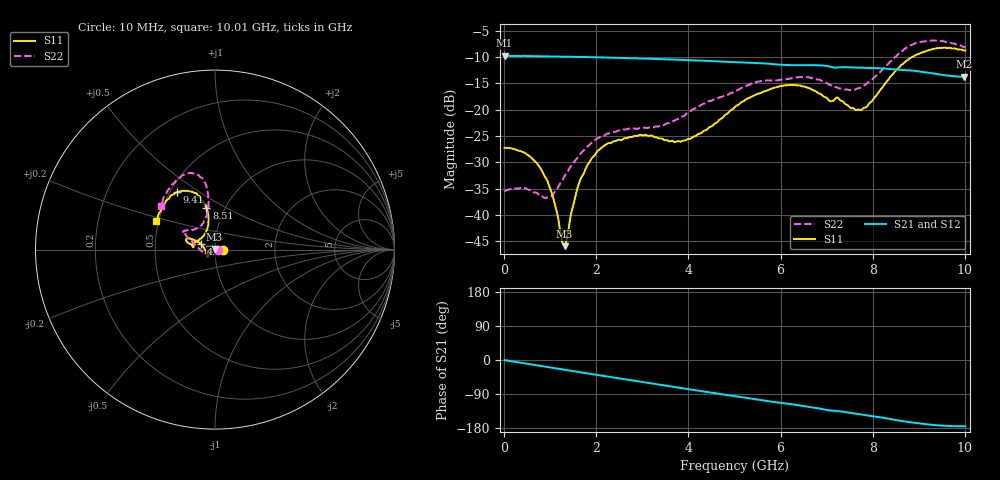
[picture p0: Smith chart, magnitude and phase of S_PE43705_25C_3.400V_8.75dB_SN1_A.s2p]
! Device ID: PE43705
! Serial: 1
! Insertion: A
! Impedance: 50 ohm
! Temp: 25C
! VDD: 3.400V
! Attenuation Step: 8.75dB
#  Hz  S  RI  R  50
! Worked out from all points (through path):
!   401 points, 10 MHz to 10.01 GHz, reference 50 ohm
!   highest |S21| = -9.78 dB at 10 MHz (marker M1); lowest = -13.8 dB at 9.985 GHz (marker M2)
!   group delay of S21, straight-line fit = 50.4 ps
!   lowest |S11| = -45.9 dB at 1.31 GHz (marker M3), VSWR 1.01, Z = 49.7 + j0.422 ohm
!   |S11| at or under -10 dB: start of sweep to 8.858 GHz
!   |S22| runs from -36.8 to -6.9 dB; largest |S21 - S12| = 0.003
!   S11 on the Smith chart (normalised r, x): 10 MHz: 1.09, +0.00; 4.76 GHz: 0.85, +0.06; 8.51 GHz: 0.82, +0.40; 9.41 GHz: 0.54, +0.41; 10.01 GHz: 0.49, +0.18
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1e7  0.0435 3.5e-06  0.3244 -0.00145  0.3246 -0.00137  0.017 0.000218
4.35e8  0.0373 0.0113  0.3193 -0.0494  0.3183 -0.0486  0.0131 0.0123
7.85e8  0.0237 0.0147  0.3089 -0.086  0.3088 -0.0857  0.00143 0.0149
1.01e9  0.0125 0.012  0.3001 -0.1094  0.3001 -0.1091  -0.00825 0.0122
1.26e9  0.000151 0.00551  0.2887 -0.1333  0.2889 -0.1331  -0.02 0.00681
1.31e9  -0.00275 0.00424  0.2863 -0.1381  0.2864 -0.1378  -0.0227 0.00567
1.685e9  -0.0207 -0.0103  0.2647 -0.1719  0.2647 -0.1718  -0.0389 -0.00648
2.21e9  -0.0355 -0.0302  0.2278 -0.2133  0.2278 -0.2132  -0.054 -0.0214
2.935e9  -0.0414 -0.0397  0.1666 -0.2567  0.167 -0.2567  -0.0631 -0.0206
3.36e9  -0.0406 -0.0345  0.1273 -0.2732  0.1277 -0.273  -0.0676 -0.0151
3.985e9  -0.052 -0.00747  0.0672 -0.2872  0.0677 -0.2868  -0.0927 0.00777
4.76e9  -0.0789 0.0325  -0.00498 -0.2848  -0.00452 -0.2848  -0.1265 0.0453
5.01e9  -0.0961 0.045  -0.0272 -0.2803  -0.0269 -0.2804  -0.1391 0.0563
5.985e9  -0.1547 0.0621  -0.1034 -0.2457  -0.1022 -0.246  -0.1663 0.0934
6.685e9  -0.1494 0.0378  -0.1509 -0.2162  -0.151 -0.2162  -0.1684 0.1056
7.71e9  -0.0688 0.0721  -0.2 -0.1501  -0.1991 -0.1502  -0.0679 0.1452
8.36e9  -0.0376 0.1953  -0.2211 -0.1014  -0.2201 -0.1027  -0.0363 0.2775
8.51e9  -0.0476 0.2314  -0.223 -0.0873  -0.2217 -0.0893  -0.0403 0.3187
8.935e9  -0.1039 0.3136  -0.2256 -0.0558  -0.2241 -0.0547  -0.096 0.417
9.41e9  -0.21 0.3202  -0.2151 -0.0283  -0.2142 -0.0281  -0.1824 0.4144
9.985e9  -0.3201 0.1698  -0.2039 -0.0186  -0.2049 -0.0191  -0.2958 0.2563
1.001e10  -0.327 0.1604  -0.2047 -0.0181  -0.206 -0.0195  -0.3028 0.2453
